{attribute 'qualified_only'}
VAR_GLOBAL CONSTANT
	(* Move types more fully in TMI documentation *)
	ABSOLUTE:UDINT := 0;
	INCREMENTAL_POSITIVE:UDINT := 1;
	INCREMENTAL_NEGATIVE:UDINT := 2;
	HOME:UDINT := 5;
	NO_ACTION:UDINT := 6;
	FORCE:UDINT := 9;
	ROTARY_INCREMENTAL_POSITIVE:UDINT := 11;
	ROTARY_INCREMENTAL_NEGATIVE:UDINT := 12;
	ROTARY_VELOCITY_FWD:UDINT :=13;
	ROTARY_VELOCITY_REV:UDINT :=14;
END_VAR
